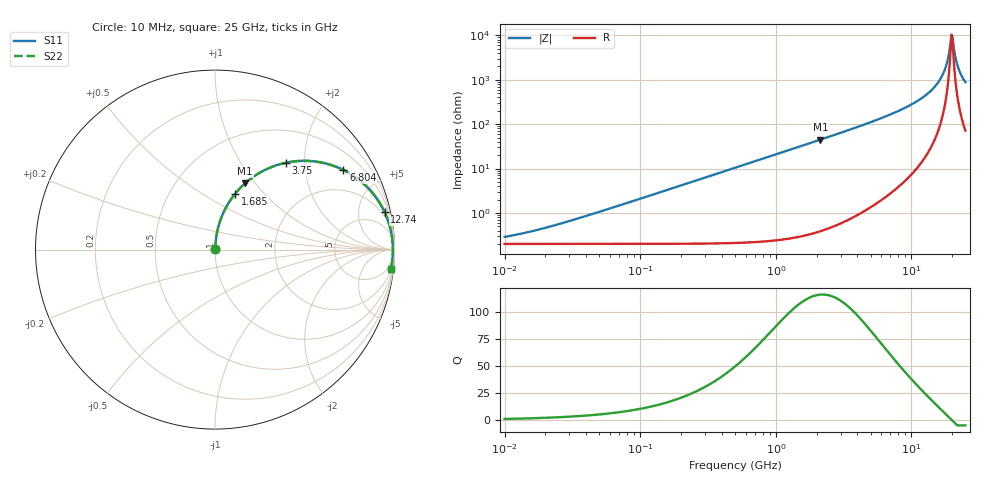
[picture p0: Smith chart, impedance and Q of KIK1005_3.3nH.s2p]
!version-3
!date-01.2023
!Series
# Hz S RI R 50
!Freq ReS11 ImS11 ReS21 ImS21 ReS12 ImS12 ReS22 ImS22
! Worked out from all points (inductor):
!   500 points, 10 MHz to 25 GHz, reference 50 ohm
!   read as one part in series: L = 3.3 nH near 29.04 MHz
!   highest Q = 116 at 2.132 GHz (marker M1), where L = 3.34 nH
!   self-resonance near 19.76 GHz
!   S11 on the Smith chart (normalised r, x): 10 MHz: 1.00, +0.00; 1.685 GHz: 1.01, +0.70; 3.75 GHz: 1.02, +1.61; 6.804 GHz: 1.05, +3.20; 12.74 GHz: 1.38, +8.96; 25 GHz: 2, -18
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1e7  0.00199 0.00207  0.998 -0.00207  0.998 -0.00207  0.00199 0.00207
1.758498e7  0.002 0.00363  0.998 -0.00363  0.998 -0.00363  0.002 0.00363
3.732484e7  0.00205 0.00771  0.998 -0.00771  0.998 -0.00771  0.00205 0.00771
1.37147e8  0.0028 0.0283  0.9972 -0.0283  0.9972 -0.0283  0.0028 0.0283
5.039353e8  0.0128 0.103  0.9872 -0.103  0.9872 -0.103  0.0128 0.103
1.685412e9  0.1124 0.3114  0.8876 -0.3114  0.8876 -0.3114  0.1124 0.3114
1.851668e9  0.1326 0.3348  0.8674 -0.3348  0.8674 -0.3348  0.1326 0.3348
2.132302e9  0.1688 0.3703  0.8312 -0.3703  0.8312 -0.3703  0.1688 0.3703
3.749649e9  0.3949 0.4839  0.6051 -0.4839  0.6051 -0.4839  0.3949 0.4839
6.803801e9  0.7155 0.4432  0.2845 -0.4432  0.2845 -0.4432  0.7155 0.4432
9.758208e9  0.8705 0.3233  0.1295 -0.3233  0.1295 -0.3233  0.8705 0.3233
1.273889e10  0.9447 0.2086  0.0553 -0.2086  0.0553 -0.2086  0.9447 0.2086
1.490138e10  0.9717 0.1362  0.0283 -0.1362  0.0283 -0.1362  0.9717 0.1362
1.689283e10  0.9848 0.0771  0.0152 -0.0771  0.0152 -0.0771  0.9848 0.0771
1.827048e10  0.9893 0.0398  0.0107 -0.0398  0.0107 -0.0398  0.9893 0.0398
1.945306e10  0.9908 0.00992  0.00918 -0.00992  0.00918 -0.00992  0.9908 0.00992
1.976048e10  0.9909 0.00245  0.00909 -0.00245  0.00909 -0.00245  0.9909 0.00245
2.038997e10  0.9908 -0.0125  0.00923 0.0125  0.00923 0.0125  0.9908 -0.0125
2.137199e10  0.9897 -0.0349  0.0103 0.0349  0.0103 0.0349  0.9897 -0.0349
2.240132e10  0.9876 -0.0573  0.0124 0.0573  0.0124 0.0573  0.9876 -0.0573
2.385127e10  0.9832 -0.0871  0.0168 0.0871  0.0168 0.0871  0.9832 -0.0871
2.5e10  0.9788 -0.1093  0.0212 0.1093  0.0212 0.1093  0.9788 -0.1093
